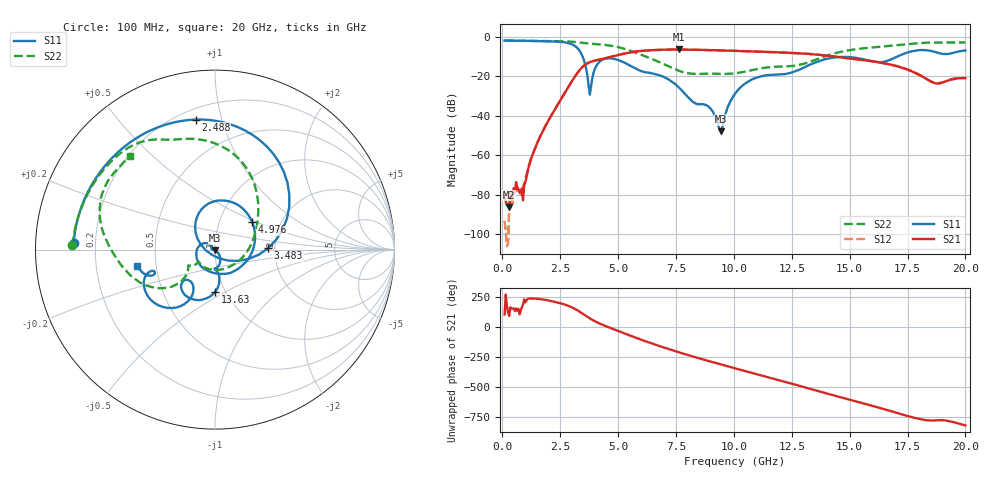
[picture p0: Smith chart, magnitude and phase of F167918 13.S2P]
!  2-Port S-parameters saved by WinCal
! VAR MeasName=S-Parameters (CALIBRATED_DATA) read from VNA (N5242A)
! VAR MeasDate=2016-11-22 10:25:26
! VAR NAME=F167918 13
! VAR FILENAME=F167918 13.S2P
! VAR DATE=2016-11-22 10:25:26
! VAR PHYS_PORTS=1,2
# Hz S DB R 50
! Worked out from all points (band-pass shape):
!   401 points, 100 MHz to 20 GHz, reference 50 ohm
!   highest |S21| = -6.58 dB at 7.612 GHz (marker M1); lowest = -86.2 dB at 299 MHz (marker M2)
!   |S21| within 3 dB of the highest: 4.929 GHz to 13.9 GHz (8.972 GHz wide, 95.3 % of centre)
!   lowest |S11| = -47.9 dB at 9.453 GHz (marker M3), VSWR 1.01, Z = 49.9 - j0.395 ohm
!   |S11| at or under -10 dB: 3.462 GHz to 17.09 GHz (13.63 GHz wide, 133 % of centre)
!   |S22| runs from -19.0 to -2.0 dB; largest |S21 - S12| = 0.0045
!   S11 on the Smith chart (normalised r, x): 100 MHz: 0.12, +0.02; 2.488 GHz: 0.26, +0.83; 3.483 GHz: 1.84, +0.03; 4.976 GHz: 1.43, +0.47; 13.63 GHz: 0.90, -0.44; 20 GHz: 0.39, -0.09
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1e8  -2.07 177.3  -80.80 103.8  -93.36 90.2  -2.00 178.3
2.99e8  -2.09 172.0  -86.22 91.6  -86.69 176.6  -2.03 175.1
8.96e8  -2.18 156.0  -82.89 -173.7  -75.72 -173.2  -2.13 165.8
1.493e9  -2.29 138.5  -54.30 -125.6  -54.38 -125.5  -2.22 156.4
2.488e9  -2.70 98.5  -32.60 -161.5  -32.62 -162.0  -2.40 139.0
3.43325e9  -9.21 9.3  -15.75 115.2  -15.75 115.2  -3.16 118.0
3.483e9  -10.56 1.5  -15.19 108.8  -15.17 108.7  -3.24 117.0
3.7815e9  -29.42 -122.5  -12.99 70.7  -12.96 70.5  -3.63 111.5
4.22925e9  -12.48 108.1  -11.58 26.1  -11.57 25.8  -4.01 101.5
4.9755e9  -11.77 36.4  -9.45 -31.6  -9.46 -31.9  -5.31 79.0
5.871e9  -16.89 -71.0  -7.48 -97.7  -7.47 -97.8  -8.65 49.9
6.7665e9  -19.56 -171.9  -6.75 -158.3  -6.75 -158.4  -12.90 17.3
7.61225e9  -25.61 140.1  -6.58 149.5  -6.60 149.4  -17.26 -34.8
9.453e9  -47.90 -101.0  -7.03 46.4  -7.04 46.3  -18.94 -140.4
1.005e10  -28.94 -50.7  -7.22 14.6  -7.24 14.7  -18.68 -143.3
1.179125e10  -19.28 -90.2  -7.96 -76.2  -7.94 -76.1  -15.35 -148.7
1.338325e10  -13.78 -84.7  -8.95 -161.2  -8.91 -160.8  -12.39 -137.1
1.3632e10  -12.61 -89.7  -9.23 -174.6  -9.18 -174.3  -11.30 -137.1
1.51245e10  -10.55 -127.3  -11.29 107.2  -11.22 107.2  -6.68 -157.7
1.67165e10  -11.96 -118.3  -14.08 20.9  -14.03 21.2  -4.70 179.4
1.87065e10  -7.88 -160.2  -23.67 -59.7  -23.56 -60.2  -3.02 149.4
2e10  -7.07 -168.1  -21.07 -101.9  -20.95 -102.6  -3.04 132.5
